(* Logix 5000 AddOnInstructionDefinition export SPEL_BaseGet; software revision 30.01 *)

ADD_ON_INSTRUCTION SPEL_ExecCmd   (* revision 1.2 *)
// Executes a command in the robot controller.  Normally this is called by higher level AOIs.
VAR_INPUT
   Start : BOOL; {required}
   MaxTime : DINT := 3000; {required}
END_VAR
VAR_OUTPUT
   InCycle : BOOL; {access Read Only, visible}
   Done : BOOL; {access Read Only, visible}
   Error : BOOL; {access Read Only, visible}
END_VAR
VAR_IN_OUT
   ExtInputs : AB:ETHERNET_MODULE_INT_128Bytes:I:0; {required}
        .DATA[0].0   // ExtCmdGet
        .DATA[0].1   // ExtRespSet
        .DATA[0].2   // ExtCmdResult
        .DATA[0].3   // ExtError
   ExtOutputs : AB:ETHERNET_MODULE_INT_128Bytes:O:0; {required}
        .DATA[0].0   // ExtCmdSet
        .DATA[0].1   // ExtRespGet
        .DATA[0].2   // ExtCmdReset
END_VAR
VAR_INPUT
   Cmd : INT; {required}
   CmdParam1 : INT; {required}
   CmdParam2 : INT; {required}
   CmdParam3 : INT; {required}
   CmdParam4 : INT; {required}
   CmdParam5 : INT; {required}
   CmdParam6 : INT; {required}
   CmdParam7 : INT; {required}
END_VAR
VAR_OUTPUT
   CmdEcho : INT; {access Read Only, visible}
   Resp1 : INT; {access Read Only, visible}
   Resp2 : INT; {access Read Only, visible}
   Resp3 : INT; {access Read Only, visible}
   Resp4 : INT; {access Read Only, visible}
   Resp5 : INT; {access Read Only, visible}
   Resp6 : INT; {access Read Only, visible}
   Resp7 : INT; {access Read Only, visible}
   ErrCode1 : INT; {access Read Only, visible}
   ErrCode2 : INT; {access Read Only, visible}
END_VAR
VAR
   ExtReset : BOOL; {access None}
   ExtError : BOOL; {access None}
   ExtCmdSet : BOOL; {access None}   // Cmd Ready
   ExtCmdGet : BOOL; {access None}   // Cmd Received
   CmdXferDone : BOOL; {access None}
   ExtRespSet : BOOL; {access None}   // Resp Ready
   RespXferDone : BOOL; {access None}
   ExtCmdResult : BOOL; {access None}   // Normal or Error?
   TmrCmdDataRdy : TIMER := (PRE := 5); {access None}
   OneShotDoneOff : BOOL; {access None}
   OneShotStart : BOOL; {access None}
   StartInit : BOOL; {access None}
   OneShotStartError : BOOL; {access None}
   TmrCycle : TIMER := (PRE := 5000); {access None}
   OneshotTmrPreset : BOOL; {access None}
   TmrCmdSet : TIMER := (PRE := 20); {access None}
   OnShotCmdDataXfer : BOOL; {access None}
   OneShotRespDataXfer : BOOL; {access None}
   OneShotDataRdy : BOOL; {access None}
   OtherCmdInCycle : BOOL; {access None}
   s : BOOL; {access None}
   OneShotUnsetCmdIncycle : BOOL; {access None}
   OneShotSetCmdIncycle : BOOL; {access None}
   OneShotSetOtherCmdInCycleError : BOOL; {access None}
   OneShotSetBit : BOOL; {access None}
   MaxTimeError : BOOL; {access None}
END_VAR

ROUTINE Logic   (* ladder *)
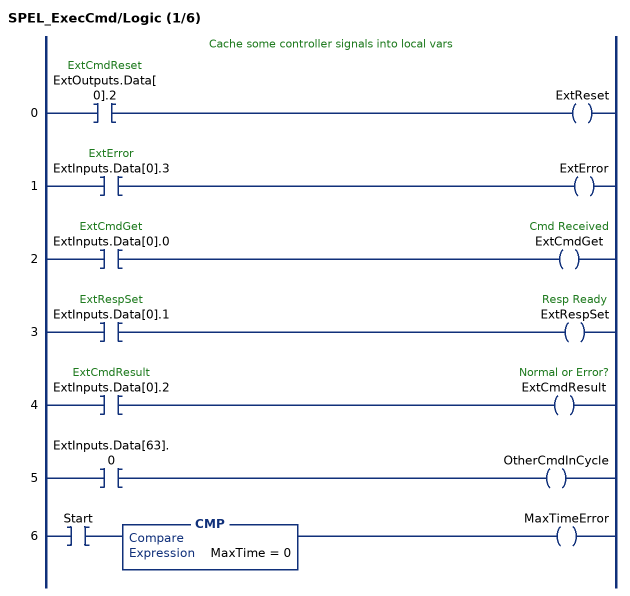
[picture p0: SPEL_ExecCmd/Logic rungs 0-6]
   // Cache some controller signals into local vars
   0: XIC(ExtOutputs.Data[0].2)OTE(ExtReset);
   1: XIC(ExtInputs.Data[0].3)OTE(ExtError);
   2: XIC(ExtInputs.Data[0].0)OTE(ExtCmdGet);
   3: XIC(ExtInputs.Data[0].1)OTE(ExtRespSet);
   4: XIC(ExtInputs.Data[0].2)OTE(ExtCmdResult);
   5: XIC(ExtInputs.Data[63].0)OTE(OtherCmdInCycle);
   6: XIC(Start)CMP(MaxTime = 0)OTE(MaxTimeError);
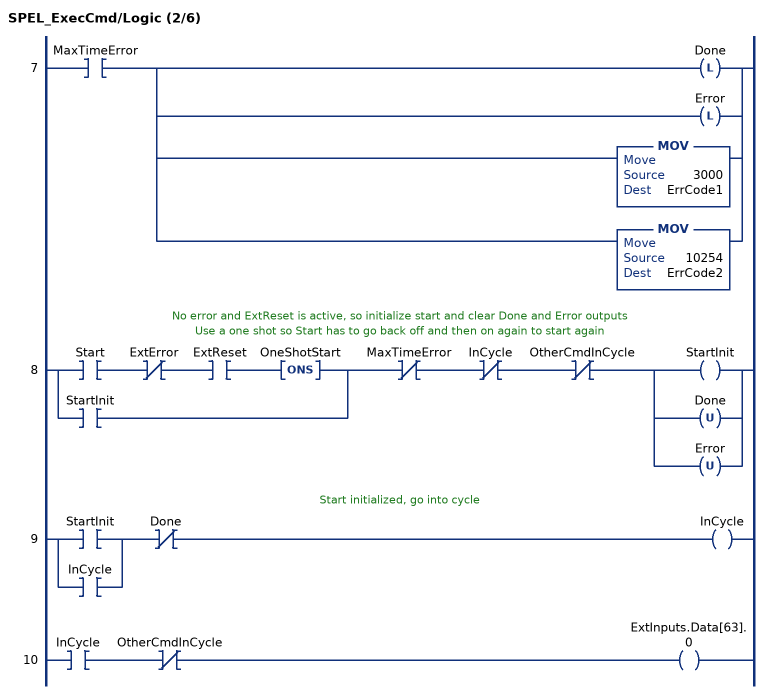
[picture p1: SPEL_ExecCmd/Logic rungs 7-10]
   7: XIC(MaxTimeError)[OTL(Done) ,OTL(Error) ,MOV(3000,ErrCode1) ,MOV(10254,ErrCode2) ];
   // No error and ExtReset is active, so initialize start and clear Done and Error outputs
   // Use a one shot so Start has to go back off and then on again to start again
   8: [XIC(Start) XIO(ExtError) XIC(ExtReset) ONS(OneShotStart) ,XIC(StartInit) ]XIO(MaxTimeError)XIO(InCycle)XIO(OtherCmdInCycle)[OTE(StartInit) ,OTU(Done) ,OTU(Error) ];
   // Start initialized, go into cycle
   9: [XIC(StartInit) ,XIC(InCycle) ]XIO(Done)OTE(InCycle);
   10: XIC(InCycle)XIO(OtherCmdInCycle)OTE(ExtInputs.Data[63].0);
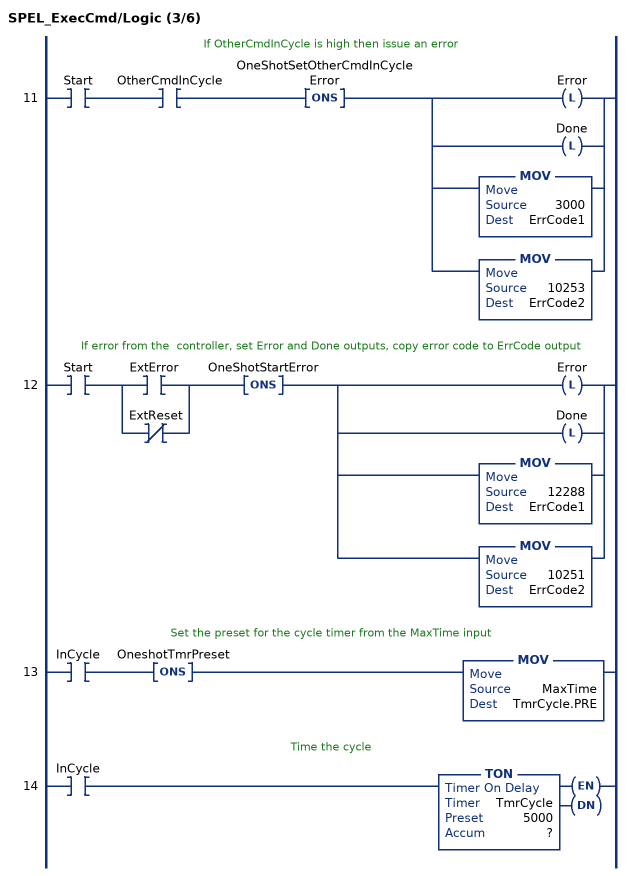
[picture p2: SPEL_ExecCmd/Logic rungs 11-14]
   // If OtherCmdInCycle is high then issue an error
   11: XIC(Start)XIC(OtherCmdInCycle)ONS(OneShotSetOtherCmdInCycleError)[OTL(Error) ,OTL(Done) ,MOV(3000,ErrCode1) ,MOV(10253,ErrCode2) ];
   // If error from the  controller, set Error and Done outputs, copy error code to ErrCode output
   12: XIC(Start)[XIC(ExtError) ,XIO(ExtReset) ]ONS(OneShotStartError)[OTL(Error) ,OTL(Done) ,MOV(12288,ErrCode1) ,MOV(10251,ErrCode2) ];
   // Set the preset for the cycle timer from the MaxTime input
   13: XIC(InCycle)ONS(OneshotTmrPreset)MOV(MaxTime,TmrCycle.PRE);
   // Time the cycle
   14: XIC(InCycle)TON(TmrCycle,?,?);
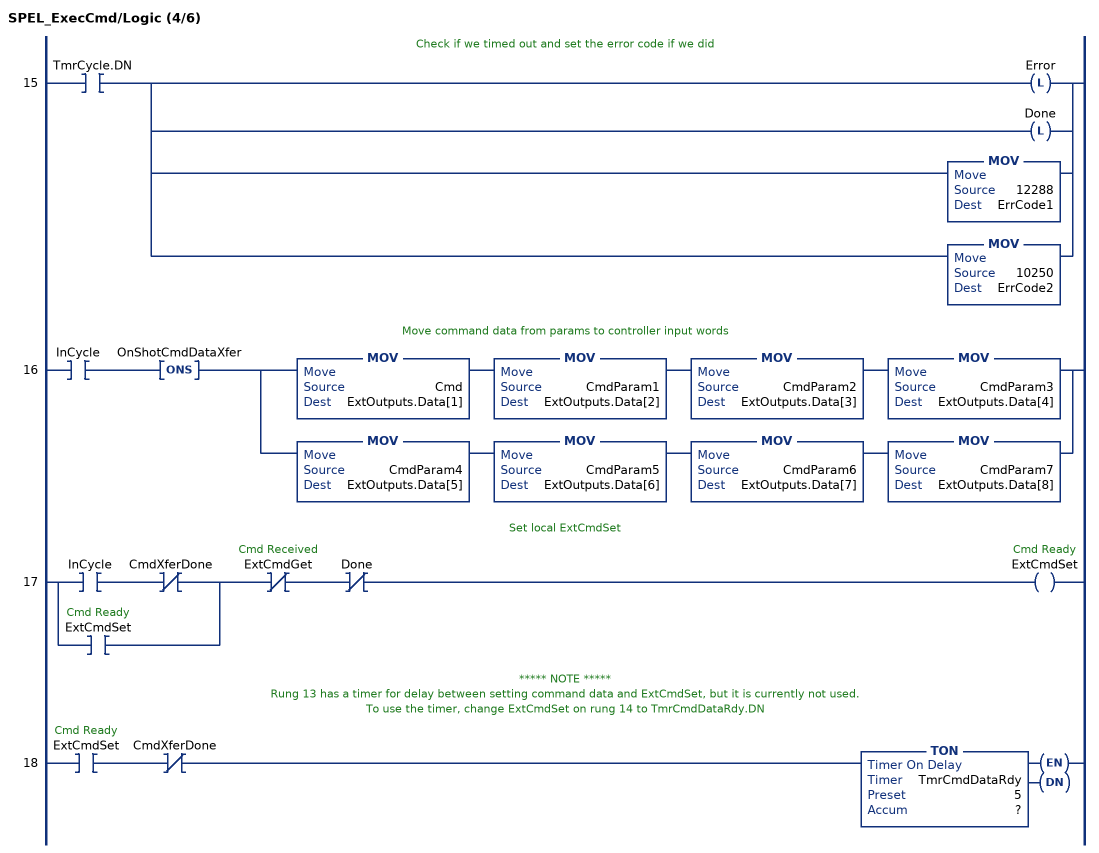
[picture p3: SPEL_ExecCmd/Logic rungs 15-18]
   // Check if we timed out and set the error code if we did
   15: XIC(TmrCycle.DN)[OTL(Error) ,OTL(Done) ,MOV(12288,ErrCode1) ,MOV(10250,ErrCode2) ];
   // Move command data from params to controller input words
   16: XIC(InCycle)ONS(OnShotCmdDataXfer)[MOV(Cmd,ExtOutputs.Data[1]) MOV(CmdParam1,ExtOutputs.Data[2]) MOV(CmdParam2,ExtOutputs.Data[3]) MOV(CmdParam3,ExtOutputs.Data[4]) ,MOV(CmdParam4,ExtOutputs.Data[5]) MOV(CmdParam5,ExtOutputs.Data[6]) MOV(CmdParam6,ExtOutputs.Data[7]) MOV(CmdParam7,ExtOutputs.Data[8]) ];
   // Set local ExtCmdSet
   17: [XIC(InCycle) XIO(CmdXferDone) ,XIC(ExtCmdSet) ]XIO(ExtCmdGet)XIO(Done)OTE(ExtCmdSet);
   // ***** NOTE *****
   // Rung 13 has a timer for delay between setting command data and ExtCmdSet, but it is currently not used.
   // To use the timer, change ExtCmdSet on rung 14 to TmrCmdDataRdy.DN
   18: XIC(ExtCmdSet)XIO(CmdXferDone)TON(TmrCmdDataRdy,?,?);
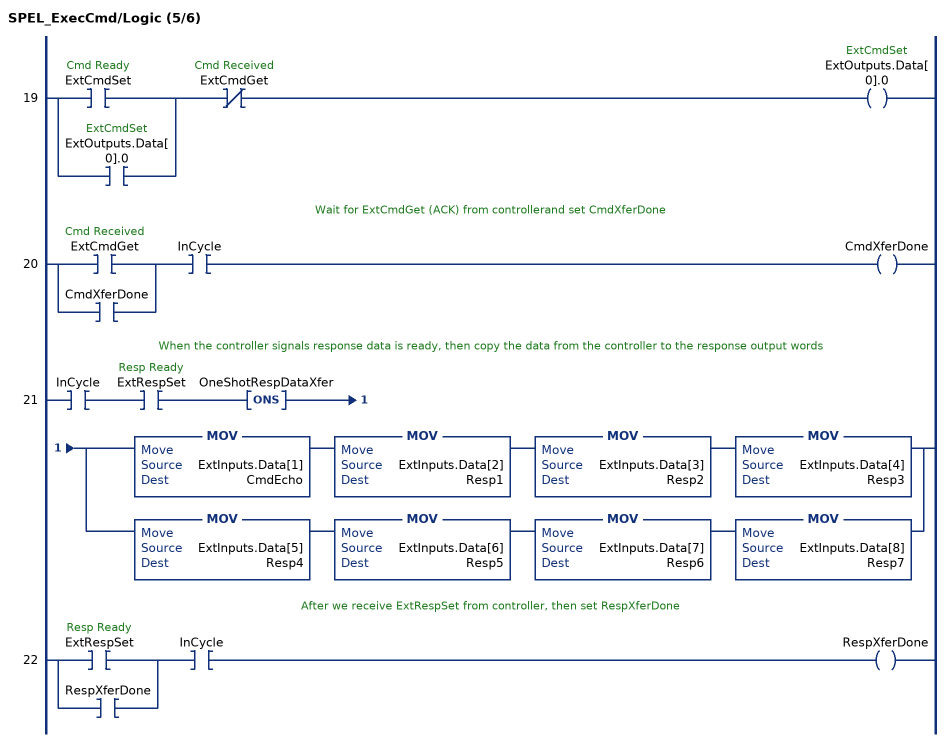
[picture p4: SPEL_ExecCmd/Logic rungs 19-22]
   19: [XIC(ExtCmdSet) ,XIC(ExtOutputs.Data[0].0) ]XIO(ExtCmdGet)OTE(ExtOutputs.Data[0].0);
   // Wait for ExtCmdGet (ACK) from controllerand set CmdXferDone
   20: [XIC(ExtCmdGet) ,XIC(CmdXferDone) ]XIC(InCycle)OTE(CmdXferDone);
   // When the controller signals response data is ready, then copy the data from the controller to the response output words
   21: XIC(InCycle)XIC(ExtRespSet)ONS(OneShotRespDataXfer)[MOV(ExtInputs.Data[1],CmdEcho) MOV(ExtInputs.Data[2],Resp1) MOV(ExtInputs.Data[3],Resp2) MOV(ExtInputs.Data[4],Resp3) ,MOV(ExtInputs.Data[5],Resp4) MOV(ExtInputs.Data[6],Resp5) MOV(ExtInputs.Data[7],Resp6) MOV(ExtInputs.Data[8],Resp7) ];
   // After we receive ExtRespSet from controller, then set RespXferDone
   22: [XIC(ExtRespSet) ,XIC(RespXferDone) ]XIC(InCycle)OTE(RespXferDone);
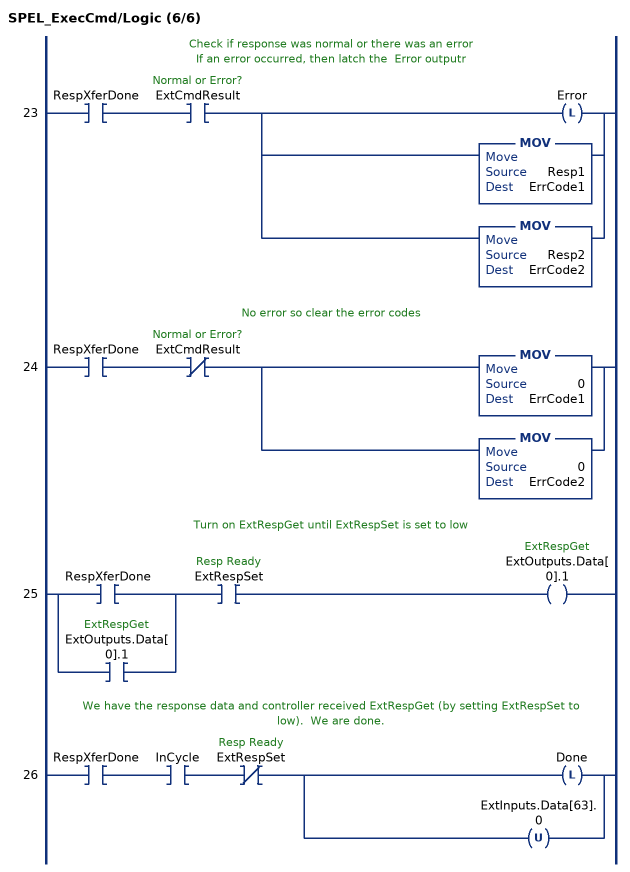
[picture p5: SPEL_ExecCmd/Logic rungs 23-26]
   // Check if response was normal or there was an error
   // If an error occurred, then latch the  Error outputr
   23: XIC(RespXferDone)XIC(ExtCmdResult)[OTL(Error) ,MOV(Resp1,ErrCode1) ,MOV(Resp2,ErrCode2) ];
   // No error so clear the error codes
   24: XIC(RespXferDone)XIO(ExtCmdResult)[MOV(0,ErrCode1) ,MOV(0,ErrCode2) ];
   // Turn on ExtRespGet until ExtRespSet is set to low
   25: [XIC(RespXferDone) ,XIC(ExtOutputs.Data[0].1) ]XIC(ExtRespSet)OTE(ExtOutputs.Data[0].1);
   // We have the response data and controller received ExtRespGet (by setting ExtRespSet to low).  We are done.
   26: XIC(RespXferDone)XIC(InCycle)XIO(ExtRespSet)[OTL(Done) ,OTU(ExtInputs.Data[63].0) ];
END_ROUTINE
END_ADD_ON_INSTRUCTION

ADD_ON_INSTRUCTION SPEL_BaseGet   (* revision 1.2, vendor SEIKO EPSON CORP. *)
// Gets the base coordinate system.
VAR_INPUT
   Start : BOOL; {required}
END_VAR
VAR_OUTPUT
   InCycle : BOOL; {access Read Only, visible}
   Done : BOOL; {access Read Only, visible}
   Error : BOOL; {access Read Only, visible}
END_VAR
VAR_INPUT
   NumAxes : INT; {required}
END_VAR
VAR_OUTPUT
   BaseX : REAL; {visible}
   BaseY : REAL; {visible}
   BaseZ : REAL; {visible}
   BaseU : REAL; {visible}
   BaseV : REAL; {visible}
   BaseW : REAL; {visible}
END_VAR
VAR_IN_OUT
   ExtInputs : AB:ETHERNET_MODULE_INT_128Bytes:I:0; {required}
   ExtOutputs : AB:ETHERNET_MODULE_INT_128Bytes:O:0; {required}
END_VAR
VAR_OUTPUT
   ErrCode1 : INT; {access Read Only, visible}
   ErrCode2 : INT; {access Read Only, visible}
END_VAR
VAR
   Coordinatex1000 : DINT; {access None}
   Coordinate_INTS : INT[2]; {access None}
   OneShotStart : BOOL[32]; {access None}
   StartInit : BOOL[32]; {access None}
   ExecBaseGetW : SPEL_ExecCmd := (MaxTime := 3000); {access None}
   ExecBaseGetV : SPEL_ExecCmd := (MaxTime := 3000); {access None}
   ExecBaseGetU : SPEL_ExecCmd := (MaxTime := 3000); {access None}
   ExecBaseGetZ : SPEL_ExecCmd := (MaxTime := 3000); {access None}
   ExecBaseGetY : SPEL_ExecCmd := (MaxTime := 3000); {access None}
   ExecBaseGetX : SPEL_ExecCmd := (MaxTime := 3000); {access None}
   X6 : BOOL; {access None}
   ExecTimeout : DINT := 5000; {access None}
END_VAR

ROUTINE Logic   (* ladder *)
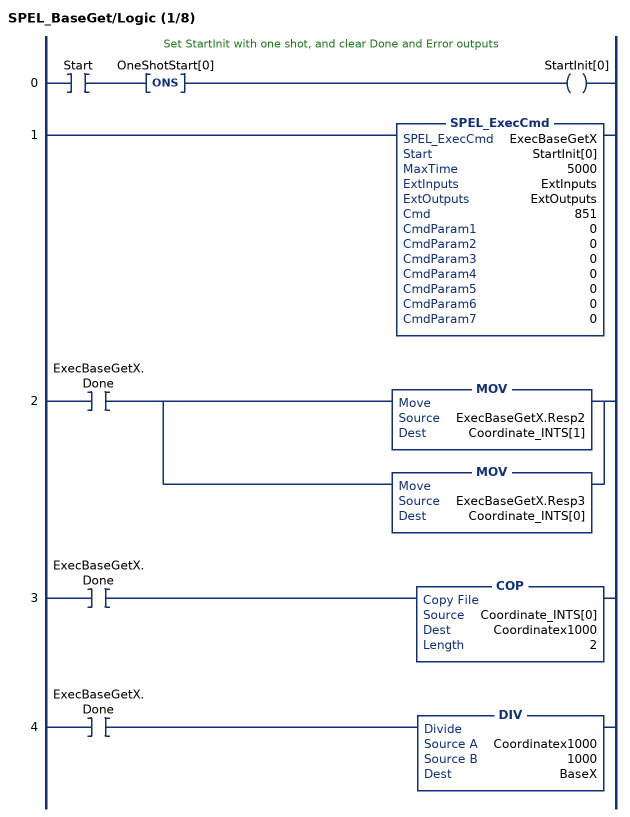
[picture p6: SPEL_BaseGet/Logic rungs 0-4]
   // Set StartInit with one shot, and clear Done and Error outputs
   0: XIC(Start)ONS(OneShotStart[0])OTE(StartInit[0]);
   1: SPEL_ExecCmd(ExecBaseGetX,StartInit[0],5000,ExtInputs,ExtOutputs,851,0,0,0,0,0,0,0);
   2: XIC(ExecBaseGetX.Done)[MOV(ExecBaseGetX.Resp2,Coordinate_INTS[1]) ,MOV(ExecBaseGetX.Resp3,Coordinate_INTS[0]) ];
   3: XIC(ExecBaseGetX.Done)COP(Coordinate_INTS[0],Coordinatex1000,2);
   4: XIC(ExecBaseGetX.Done)DIV(Coordinatex1000,1000,BaseX);
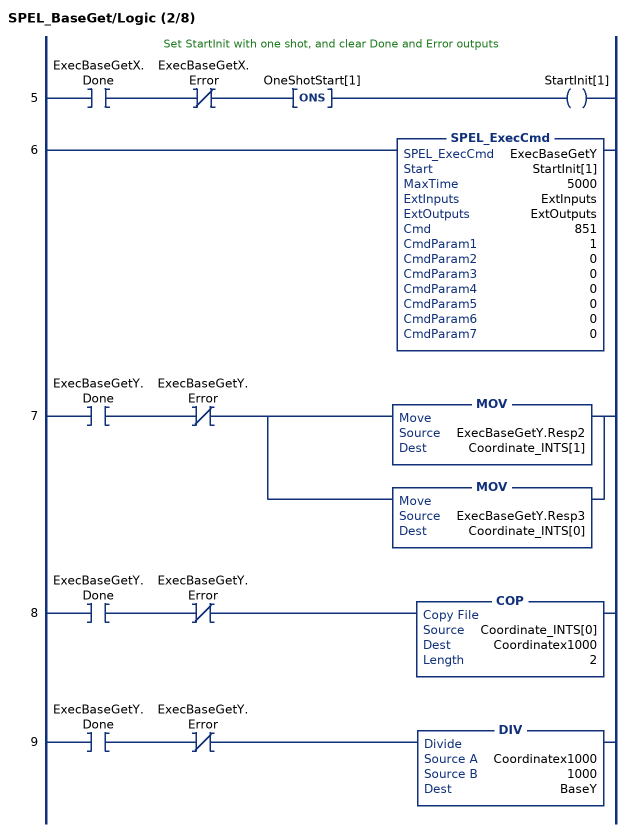
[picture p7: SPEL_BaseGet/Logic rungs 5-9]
   // Set StartInit with one shot, and clear Done and Error outputs
   5: XIC(ExecBaseGetX.Done)XIO(ExecBaseGetX.Error)ONS(OneShotStart[1])OTE(StartInit[1]);
   6: SPEL_ExecCmd(ExecBaseGetY,StartInit[1],5000,ExtInputs,ExtOutputs,851,1,0,0,0,0,0,0);
   7: XIC(ExecBaseGetY.Done)XIO(ExecBaseGetY.Error)[MOV(ExecBaseGetY.Resp2,Coordinate_INTS[1]) ,MOV(ExecBaseGetY.Resp3,Coordinate_INTS[0]) ];
   8: XIC(ExecBaseGetY.Done)XIO(ExecBaseGetY.Error)COP(Coordinate_INTS[0],Coordinatex1000,2);
   9: XIC(ExecBaseGetY.Done)XIO(ExecBaseGetY.Error)DIV(Coordinatex1000,1000,BaseY);
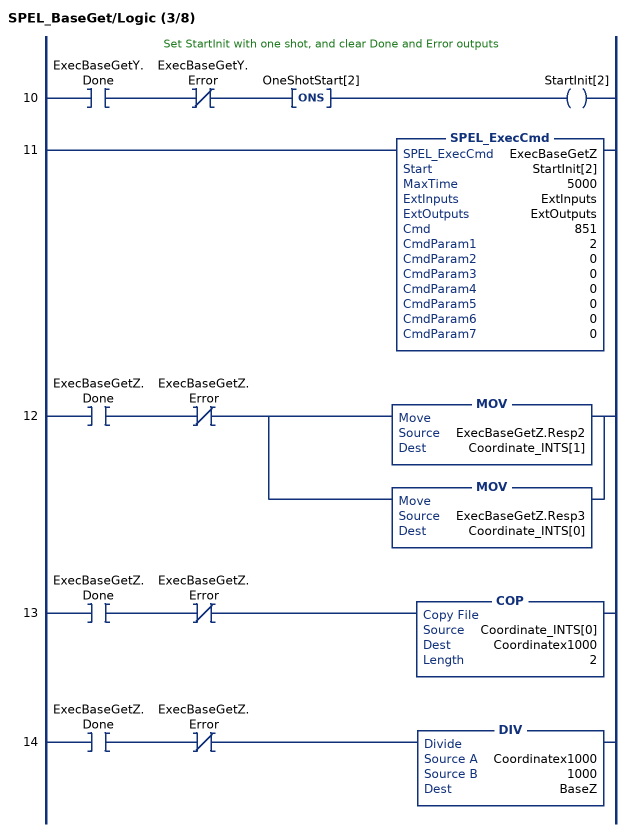
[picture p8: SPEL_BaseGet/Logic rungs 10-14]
   // Set StartInit with one shot, and clear Done and Error outputs
   10: XIC(ExecBaseGetY.Done)XIO(ExecBaseGetY.Error)ONS(OneShotStart[2])OTE(StartInit[2]);
   11: SPEL_ExecCmd(ExecBaseGetZ,StartInit[2],5000,ExtInputs,ExtOutputs,851,2,0,0,0,0,0,0);
   12: XIC(ExecBaseGetZ.Done)XIO(ExecBaseGetZ.Error)[MOV(ExecBaseGetZ.Resp2,Coordinate_INTS[1]) ,MOV(ExecBaseGetZ.Resp3,Coordinate_INTS[0]) ];
   13: XIC(ExecBaseGetZ.Done)XIO(ExecBaseGetZ.Error)COP(Coordinate_INTS[0],Coordinatex1000,2);
   14: XIC(ExecBaseGetZ.Done)XIO(ExecBaseGetZ.Error)DIV(Coordinatex1000,1000,BaseZ);
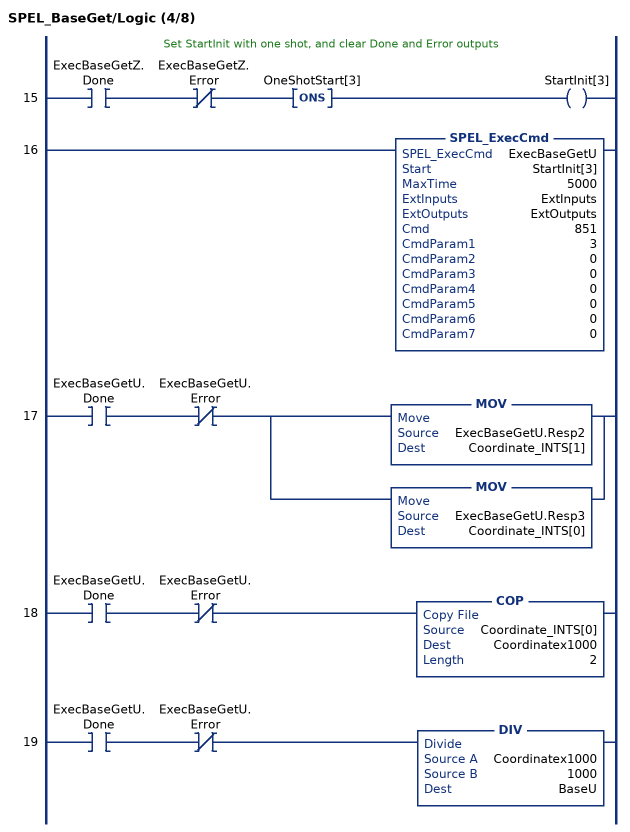
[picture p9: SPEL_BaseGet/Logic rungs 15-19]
   // Set StartInit with one shot, and clear Done and Error outputs
   15: XIC(ExecBaseGetZ.Done)XIO(ExecBaseGetZ.Error)ONS(OneShotStart[3])OTE(StartInit[3]);
   16: SPEL_ExecCmd(ExecBaseGetU,StartInit[3],5000,ExtInputs,ExtOutputs,851,3,0,0,0,0,0,0);
   17: XIC(ExecBaseGetU.Done)XIO(ExecBaseGetU.Error)[MOV(ExecBaseGetU.Resp2,Coordinate_INTS[1]) ,MOV(ExecBaseGetU.Resp3,Coordinate_INTS[0]) ];
   18: XIC(ExecBaseGetU.Done)XIO(ExecBaseGetU.Error)COP(Coordinate_INTS[0],Coordinatex1000,2);
   19: XIC(ExecBaseGetU.Done)XIO(ExecBaseGetU.Error)DIV(Coordinatex1000,1000,BaseU);
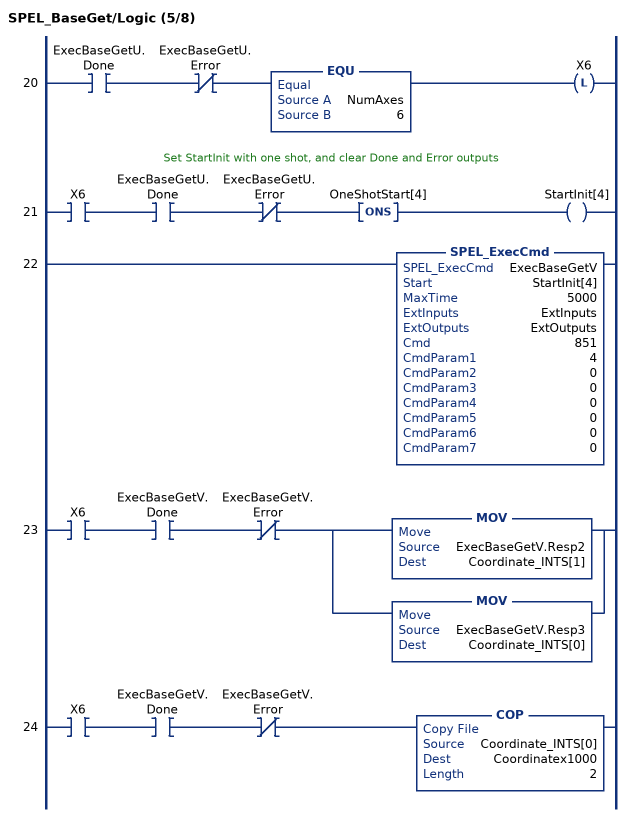
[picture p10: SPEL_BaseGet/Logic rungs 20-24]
   20: XIC(ExecBaseGetU.Done)XIO(ExecBaseGetU.Error)EQU(NumAxes,6)OTL(X6);
   // Set StartInit with one shot, and clear Done and Error outputs
   21: XIC(X6)XIC(ExecBaseGetU.Done)XIO(ExecBaseGetU.Error)ONS(OneShotStart[4])OTE(StartInit[4]);
   22: SPEL_ExecCmd(ExecBaseGetV,StartInit[4],5000,ExtInputs,ExtOutputs,851,4,0,0,0,0,0,0);
   23: XIC(X6)XIC(ExecBaseGetV.Done)XIO(ExecBaseGetV.Error)[MOV(ExecBaseGetV.Resp2,Coordinate_INTS[1]) ,MOV(ExecBaseGetV.Resp3,Coordinate_INTS[0]) ];
   24: XIC(X6)XIC(ExecBaseGetV.Done)XIO(ExecBaseGetV.Error)COP(Coordinate_INTS[0],Coordinatex1000,2);
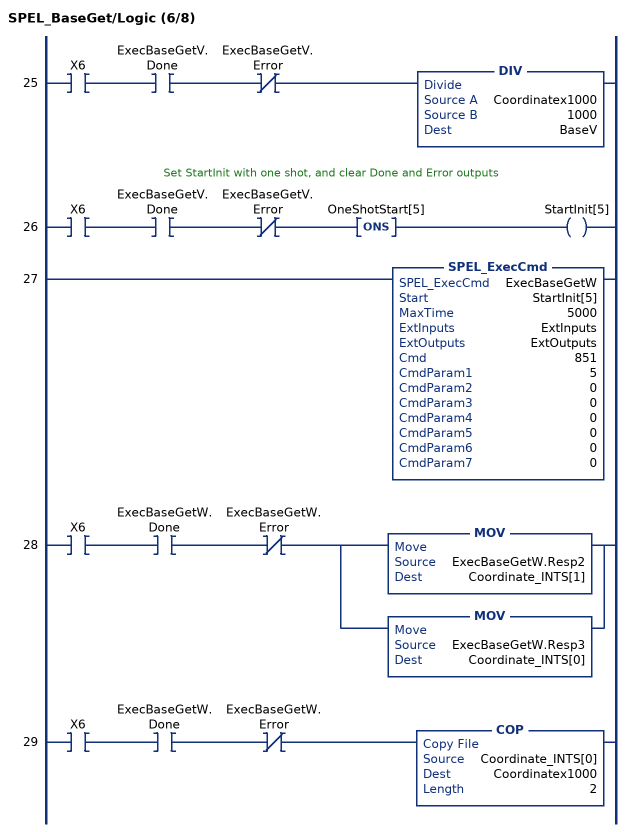
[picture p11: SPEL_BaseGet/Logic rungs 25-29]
   25: XIC(X6)XIC(ExecBaseGetV.Done)XIO(ExecBaseGetV.Error)DIV(Coordinatex1000,1000,BaseV);
   // Set StartInit with one shot, and clear Done and Error outputs
   26: XIC(X6)XIC(ExecBaseGetV.Done)XIO(ExecBaseGetV.Error)ONS(OneShotStart[5])OTE(StartInit[5]);
   27: SPEL_ExecCmd(ExecBaseGetW,StartInit[5],5000,ExtInputs,ExtOutputs,851,5,0,0,0,0,0,0);
   28: XIC(X6)XIC(ExecBaseGetW.Done)XIO(ExecBaseGetW.Error)[MOV(ExecBaseGetW.Resp2,Coordinate_INTS[1]) ,MOV(ExecBaseGetW.Resp3,Coordinate_INTS[0]) ];
   29: XIC(X6)XIC(ExecBaseGetW.Done)XIO(ExecBaseGetW.Error)COP(Coordinate_INTS[0],Coordinatex1000,2);
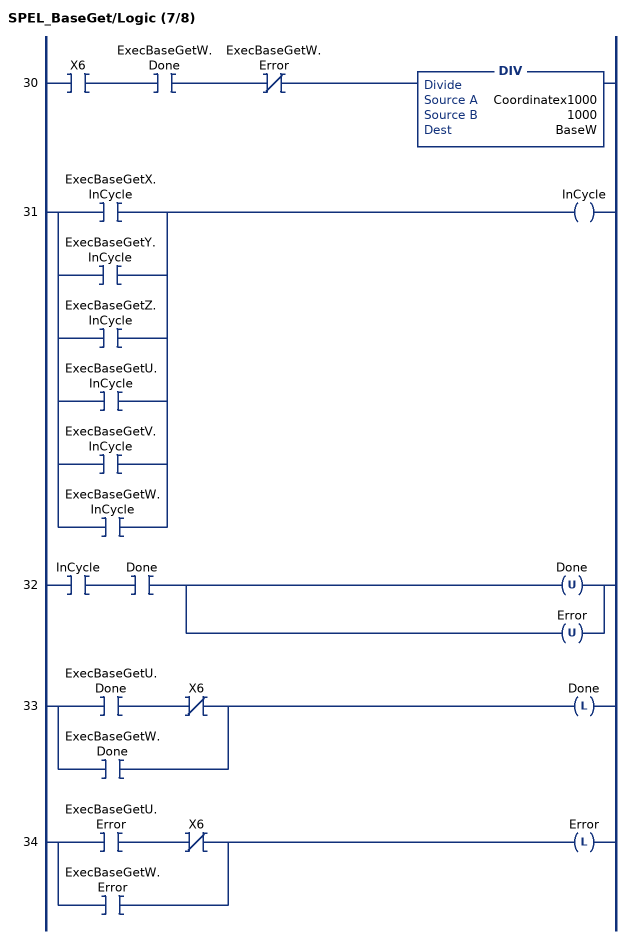
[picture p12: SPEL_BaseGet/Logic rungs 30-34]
   30: XIC(X6)XIC(ExecBaseGetW.Done)XIO(ExecBaseGetW.Error)DIV(Coordinatex1000,1000,BaseW);
   31: [XIC(ExecBaseGetX.InCycle) ,XIC(ExecBaseGetY.InCycle) ,XIC(ExecBaseGetZ.InCycle) ,XIC(ExecBaseGetU.InCycle) ,XIC(ExecBaseGetV.InCycle) ,XIC(ExecBaseGetW.InCycle) ]OTE(InCycle);
   32: XIC(InCycle)XIC(Done)[OTU(Done) ,OTU(Error) ];
   33: [XIC(ExecBaseGetU.Done) XIO(X6) ,XIC(ExecBaseGetW.Done) ]OTL(Done);
   34: [XIC(ExecBaseGetU.Error) XIO(X6) ,XIC(ExecBaseGetW.Error) ]OTL(Error);
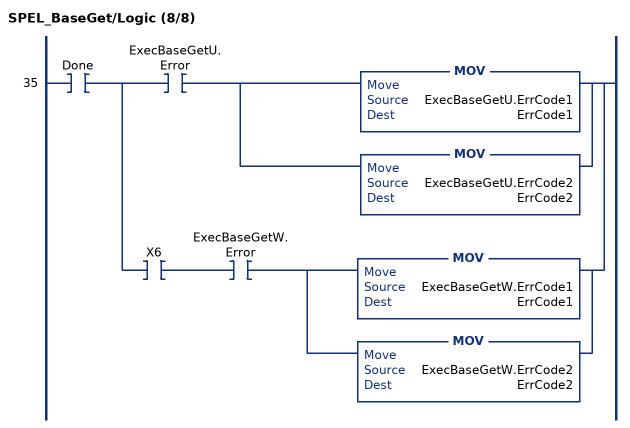
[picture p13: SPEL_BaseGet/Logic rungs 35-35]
   35: XIC(Done)[XIC(ExecBaseGetU.Error) [MOV(ExecBaseGetU.ErrCode1,ErrCode1) ,MOV(ExecBaseGetU.ErrCode2,ErrCode2) ] ,XIC(X6) XIC(ExecBaseGetW.Error) [MOV(ExecBaseGetW.ErrCode1,ErrCode1) ,MOV(ExecBaseGetW.ErrCode2,ErrCode2) ] ];
END_ROUTINE
END_ADD_ON_INSTRUCTION
